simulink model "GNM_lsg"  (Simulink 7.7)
settings: Solver=ode45  StartTime=0.0  StopTime=0.2  FixedStep=0.005  RelTol=1e-3
InitFcn:
  | GNM_lsg_ini
StopFcn:
  | GNM_lsg_plot
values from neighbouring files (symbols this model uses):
  CE = 240.02    [GNM_lsg_ini.m]
  CM = CE/2/pi    (= 38.2003694409)    [GNM_lsg_ini.m]
  Fpwm = 5000    [GNM_lsg_ini.m]
  J = 0.012    [GNM_lsg_ini.m]
  LA = 0.004    [GNM_lsg_ini.m]
  psi = 0.04    [GNM_lsg_ini.m]
  RA = 0.25    [GNM_lsg_ini.m]
  Umax = 200    [GNM_lsg_ini.m]
libraries: simulink x1

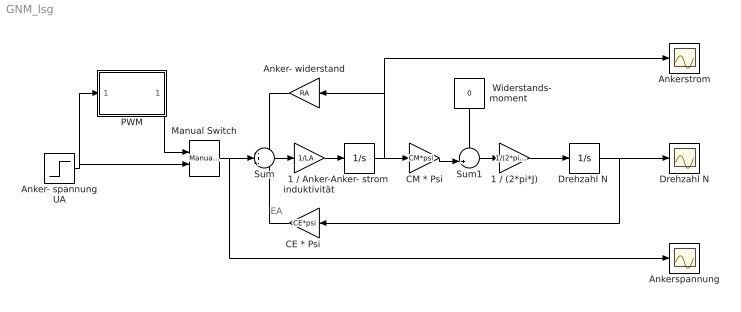
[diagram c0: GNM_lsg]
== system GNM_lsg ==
  note: EA
  " Widerstands-  moment" : Constant  Value=0
  1 / (2*pi*J) : Gain  Gain=1/(2*pi*J)
  1 / Anker- induktivität : Gain  Gain=1/LA
  Anker- spannung UA : Step  Time=0.05  After=50  SampleTime=0
  Anker- strom : Integrator
  Anker- widerstand : Gain  Gain=RA
  Ankerspannung : Scope
  Ankerstrom : Scope
  "CE * Psi " : Gain  Gain=CE*psi
  CM * Psi : Gain  Gain=CM*psi
  Drehzahl N : Scope
  "Drehzahl N " : Integrator
  Manual Switch : simulink/Signal Routing/Manual Switch  SystemSampleTime=-1  sw=0  action=0  varsize=off
  PWM : Subsystem
  Sum : Sum  Inputs=-+-
  Sum1 : Sum  Inputs=-+|
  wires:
  Anker- widerstand/1 -> Sum/1
  Anker- strom/1 -> CM * Psi/1, Anker- widerstand/1, Ankerstrom/1
  Sum/1 -> 1 / Anker- induktivität/1
  1 / Anker- induktivität/1 -> Anker- strom/1
  CM * Psi/1 -> Sum1/2
  Sum1/1 -> 1 / (2*pi*J)/1
  1 / (2*pi*J)/1 -> "Drehzahl N "/1
  " Widerstands-  moment"/1 -> Sum1/1
  "CE * Psi "/1 -> Sum/3
  "Drehzahl N "/1 -> "CE * Psi "/1, Drehzahl N/1
  Manual Switch/1 -> Sum/2, Ankerspannung/1
  PWM/1(UAist) -> Manual Switch/1
  Anker- spannung UA/1 -> PWM/1(UAsoll), Manual Switch/2

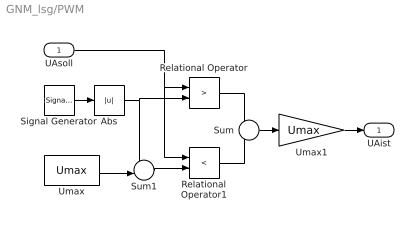
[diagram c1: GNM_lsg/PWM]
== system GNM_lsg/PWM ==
  UAsoll : Inport
  Abs : Abs
  Relational Operator : RelationalOperator  Operator=>
  Relational Operator1 : RelationalOperator  Operator=<
  Signal Generator : SignalGenerator  WaveForm=sawtooth  Amplitude=Umax  Frequency=Fpwm
  Sum : Sum  Inputs=+-
  Sum1 : Sum  Inputs=+-|
  Umax : Constant  Value=Umax
  Umax1 : Gain  Gain=Umax
  UAist : Outport  InitialOutput=0
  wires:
  Sum/1 -> Umax1/1
  Umax1/1 -> UAist/1
  Relational Operator1/1 -> Sum/2
  Relational Operator/1 -> Sum/1
  Umax/1 -> Sum1/2
  Abs/1 -> Sum1/1, Relational Operator/2
  UAsoll/1 -> Relational Operator/1, Relational Operator1/1
  Sum1/1 -> Relational Operator1/2
  Signal Generator/1 -> Abs/1
